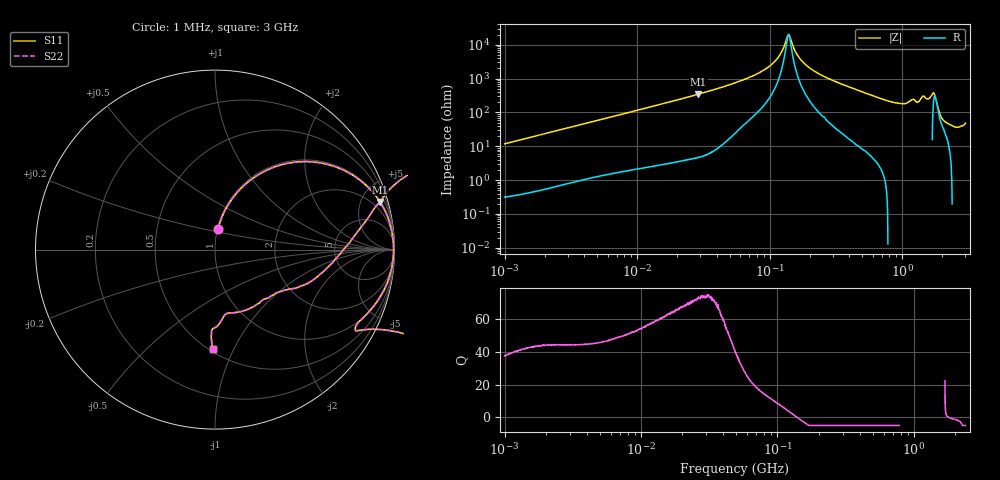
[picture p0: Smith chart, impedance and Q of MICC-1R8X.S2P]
!s-Parameter Generated by FASTRON Sdn. Bhd.
!FASTRON P/N : MICC-1R8X
!Keysight Technologies,E4991B,MY54100416,A.01.15
!Date: Fri Aug 28 09:27:39 2026
!Version  : Rev00 Fri Aug 28 09:27:39 2026
!Data & Calibration Information:
!PortZ  Port1:50+j0  Port2:50+j0
!When reading, reference impedance value at option line is always used.
!Remarks : This data is being provided solely for informational purposes.
!Freq	S11	S21	S12	S22
# Hz S dB R 50
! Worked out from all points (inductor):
!   1601 points, 1 MHz to 3 GHz, reference 50 ohm
!   read as one part in series: L = 1.87 uH near 1.041 MHz
!   highest Q = 74 at 29.01 MHz (marker M1), where L = 1.9 uH
!   self-resonance near 138.9 MHz
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1000000  -18.69 81.8  -0.09 -6.7  -0.09 -6.7  -18.69 81.8
3804036  -7.95 65.1  -0.84 -23.6  -0.84 -23.6  -7.95 65.1
1.447069e7  -1.40 30.7  -5.84 -58.4  -5.84 -58.4  -1.40 30.7
2.90111e7  -0.38 16.1  -11.15 -73.1  -11.15 -73.1  -0.38 16.1
5.477226e7  -0.11 7.6  -17.57 -80.6  -17.57 -80.6  -0.11 7.6
1.028925e8  -0.05 2.2  -28.23 -80.5  -28.23 -80.5  -0.05 2.2
1.195584e8  -0.04 1.1  -34.07 -74.7  -34.07 -74.7  -0.04 1.1
1.389236e8  -0.04 0.0  -46.11 -1.5  -46.11 -1.5  -0.04 0.0
1.663456e8  -0.05 -1.3  -32.59 76.3  -32.59 76.3  -0.05 -1.3
2.083556e8  -0.06 -3.1  -25.39 81.5  -25.39 81.5  -0.06 -3.1
7.925923e8  -0.85 -25.0  -7.49 65.1  -7.49 65.1  -0.85 -25.0
1.080907e9  -0.70 -29.2  -6.20 66.6  -6.20 66.6  -0.70 -29.2
1.182785e9  0.62 -24.8  -6.90 86.7  -6.90 86.7  0.62 -24.8
1.307284e9  3.05 -28.1  -2.91 110.8  -2.91 110.8  3.05 -28.1
1.374365e9  3.10 -19.2  -4.64 126.6  -4.64 126.6  3.10 -19.2
1.466741e9  3.43 5.3  -6.07 -164.1  -6.07 -164.1  3.43 5.3
1.526649e9  3.12 17.3  -5.01 -130.8  -5.01 -130.8  3.12 17.3
1.589003e9  1.95 21.7  -6.18 -109.5  -6.18 -109.5  1.95 21.7
1.747494e9  -1.87 7.6  -12.87 -27.8  -12.87 -27.8  -1.87 7.6
2.000286e9  -7.14 -31.8  -3.51 20.3  -3.51 20.3  -7.14 -31.8
2.568929e9  -8.84 -79.1  -0.02 20.9  -0.02 20.9  -8.84 -79.1
3e9  -5.09 -91.3  1.26 28.8  1.26 28.8  -5.09 -91.3
